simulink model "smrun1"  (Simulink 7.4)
settings: Solver=ode45  StartTime=0  StopTime=4  MaxStep=0.001  RelTol=1e-4  AbsTol=1e-4
InitFcn:
  | smdef1
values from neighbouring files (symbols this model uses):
  freq0 = 60    [IMabc2.m]    (also in imabcparam.m; IMabcrun0.m; IMabcrun1.m; imbar1.m = input('Frequency (Hz) [Press Enter to accept default 60] ='))
  ic = [fs0 fr0]    [imdef0vec.m]    (also in imdef1vec.m; imdef2vec.m = F; imic2.m = [phids phiqs phidr phiqr n0]'; imic3.m = [phids phiqs phidr phiqr n0]')
  L = length(t)    [fourierdec.m]    (also in IMabc2.m = [Lss  Lsr; IMabcf0.m = [Lss  Lsr; IMabcf1.m = [Lss  Lsr; IMcur0.m = [Ls  0   Lm  0)
  R = str2num(get(h,'string'))    [acttrcalc1.m]    (also in IMabc2.m = diag([Rs Rs Rs Rr Rr Rr]); IMabcf0.m = diag([Rs Rs Rs Rr Rr Rr]); IMabcf1.m = diag([Rs Rs Rs Rr Rr Rr]); IMcurf0.m = diag([Rs Rs Rr Rr]))
  Te0 = 0.75/wo*p*(Is*conj(Is)*Req)    [imdefSIvec1.m]
  V = [Vas 0 0].'    [Actac.m]    (also in acttrcalc1.m = str2num(get(h,'string')); im3d.m = eval(get(hVs,'String')); IMabc2.m = [vas vbs vcs 0 0 0]'; IMabcf0.m = [vas vbs vcs 0 0 0]')
undefined symbols (not defined in the file or in its folder): vf0

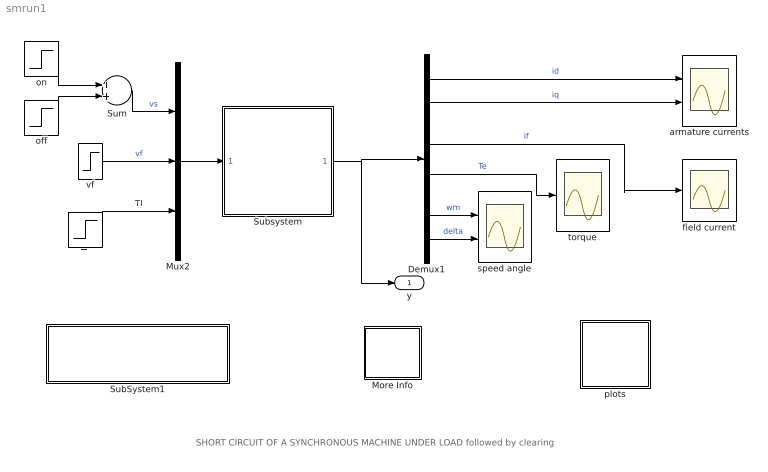
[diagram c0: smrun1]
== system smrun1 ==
  note: SHORT CIRCUIT OF A SYNCHRONOUS MACHINE UNDER LOAD followed by clearing
  Demux1 : Demux  Outputs=6
  More Info : Subsystem
  Mux2 : Mux  Inputs=3
  SubSystem1 : Subsystem
  Subsystem : Subsystem  mask{R=R, L=L, wo=2*pi*freq0, Hi=4, ic=[ic]}
      mask prompts: R "Resistance{pu]"; L "Inductance matrix [pu]"; wo "Base frequency [rad/s]"; Hi "Inertia Constant [s]"; ic "Initial Conditions"
  Sum : Sum  OutDataType=sfix(16)  OutScaling=2^0
  Tl : Step  Time=0  After=Te0  SampleTime=0
  armature currents : Scope  NumInputPorts=2
  field current : Scope
  off : Step  Time=.6  Before=0.0  After=V  SampleTime=0
  on : Step  Time=0.5  Before=V  After=0  SampleTime=0
  plots : Subsystem
  speed angle : Scope  NumInputPorts=2
  torque : Scope
  vf : Step  Time=0  After=vf0  SampleTime=0
  y : Outport
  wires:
  Demux1/3 -> field current/1  "if"
  Demux1/4 -> torque/1  "Te"
  Demux1/2 -> armature currents/2  "iq"
  Demux1/1 -> armature currents/1  "id"
  vf/1 -> Mux2/2  "vf"
  Tl/1 -> Mux2/3  "Tl"
  Sum/1 -> Mux2/1  "vs"
  on/1 -> Sum/1
  off/1 -> Sum/2
  Demux1/6 -> speed angle/2  "delta"
  Demux1/5 -> speed angle/1  "wm"
  Mux2/1 -> Subsystem/1(In1)
  Subsystem/1(Out1) -> Demux1/1, y/1

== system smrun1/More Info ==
  note: SHORT CIRCUIT OF A SYNCHRONOUS MACHINE UNDER LOAD followed by clearing

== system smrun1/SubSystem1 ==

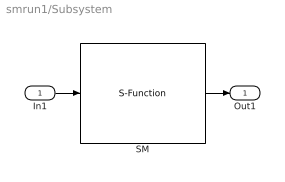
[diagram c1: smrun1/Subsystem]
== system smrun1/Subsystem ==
  In1 : Inport  OutDataType=sfix(16)  OutScaling=2^0
  SM : S-Function  FunctionName=smmod  Parameters=R,L,Hi,wo,ic  EnableBusSupport=off
  Out1 : Outport
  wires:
  SM/1 -> Out1/1
  In1/1 -> SM/1

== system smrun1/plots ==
